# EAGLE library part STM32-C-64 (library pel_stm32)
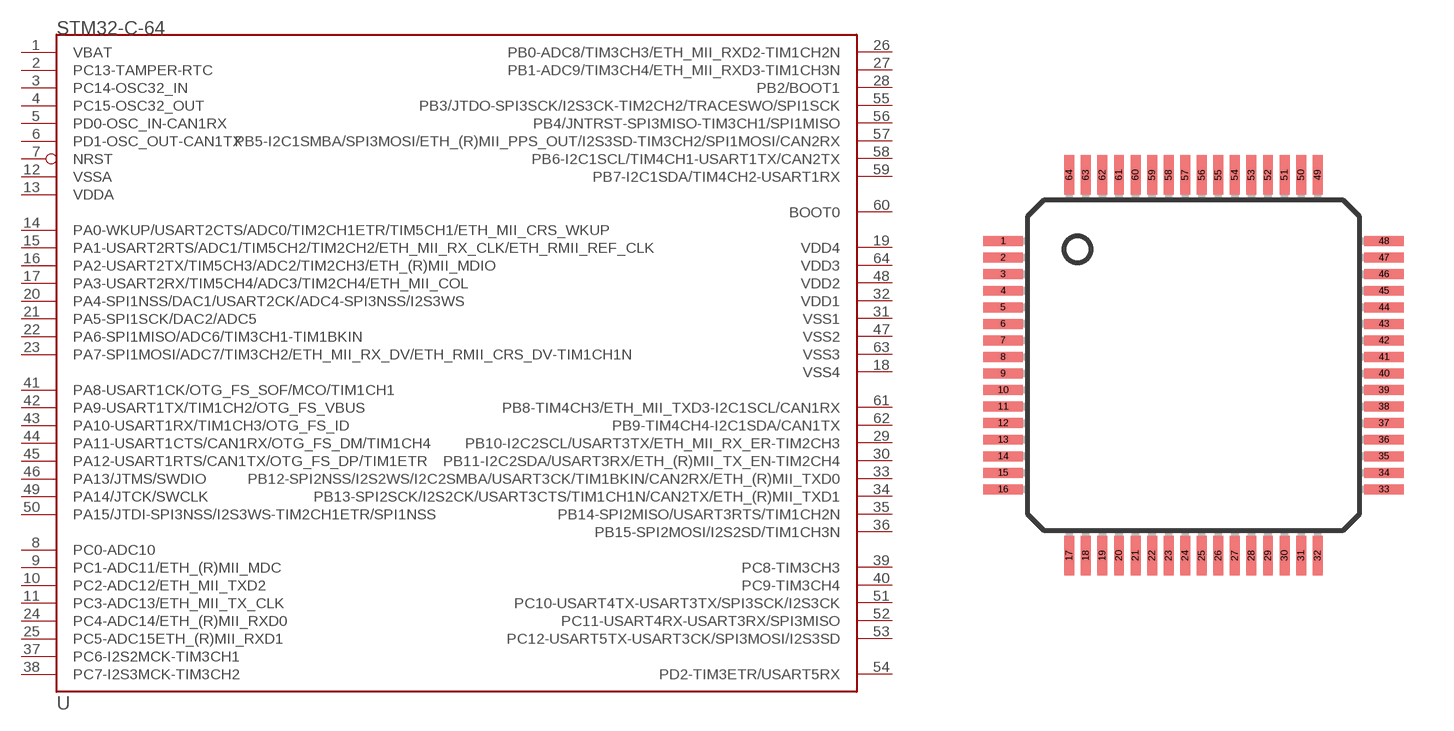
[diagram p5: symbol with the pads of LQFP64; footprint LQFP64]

Designator prefix U

## STM32-C-64  [LQFP64]
1  VBAT  sup
2  PC13-TAMPER-RTC
3  PC14-OSC32_IN
4  PC15-OSC32_OUT
5  PD0-OSC_IN-CAN1RX  in
6  PD1-OSC_OUT-CAN1TX  out
7  NRST
8  PC0-ADC10
9  PC1-ADC11/ETH_(R)MII_MDC
10  PC2-ADC12/ETH_MII_TXD2
11  PC3-ADC13/ETH_MII_TX_CLK
12  VSSA  sup
13  VDDA  sup
14  PA0-WKUP/USART2CTS/ADC0/TIM2CH1ETR/TIM5CH1/ETH_MII_CRS_WKUP
15  PA1-USART2RTS/ADC1/TIM5CH2/TIM2CH2/ETH_MII_RX_CLK/ETH_RMII_REF_CLK
16  PA2-USART2TX/TIM5CH3/ADC2/TIM2CH3/ETH_(R)MII_MDIO
17  PA3-USART2RX/TIM5CH4/ADC3/TIM2CH4/ETH_MII_COL
18  VSS4
19  VDD4
20  PA4-SPI1NSS/DAC1/USART2CK/ADC4-SPI3NSS/I2S3WS
21  PA5-SPI1SCK/DAC2/ADC5
22  PA6-SPI1MISO/ADC6/TIM3CH1-TIM1BKIN
23  PA7-SPI1MOSI/ADC7/TIM3CH2/ETH_MII_RX_DV/ETH_RMII_CRS_DV-TIM1CH1N
24  PC4-ADC14/ETH_(R)MII_RXD0
25  PC5-ADC15ETH_(R)MII_RXD1
26  PB0-ADC8/TIM3CH3/ETH_MII_RXD2-TIM1CH2N
27  PB1-ADC9/TIM3CH4/ETH_MII_RXD3-TIM1CH3N
28  PB2/BOOT1
29  PB10-I2C2SCL/USART3TX/ETH_MII_RX_ER-TIM2CH3
30  PB11-I2C2SDA/USART3RX/ETH_(R)MII_TX_EN-TIM2CH4
31  VSS1  sup
32  VDD1  sup
33  PB12-SPI2NSS/I2S2WS/I2C2SMBA/USART3CK/TIM1BKIN/CAN2RX/ETH_(R)MII_TXD0
34  PB13-SPI2SCK/I2S2CK/USART3CTS/TIM1CH1N/CAN2TX/ETH_(R)MII_TXD1
35  PB14-SPI2MISO/USART3RTS/TIM1CH2N
36  PB15-SPI2MOSI/I2S2SD/TIM1CH3N
37  PC6-I2S2MCK-TIM3CH1
38  PC7-I2S3MCK-TIM3CH2
39  PC8-TIM3CH3
40  PC9-TIM3CH4
41  PA8-USART1CK/OTG_FS_SOF/MCO/TIM1CH1
42  PA9-USART1TX/TIM1CH2/OTG_FS_VBUS
43  PA10-USART1RX/TIM1CH3/OTG_FS_ID
44  PA11-USART1CTS/CAN1RX/OTG_FS_DM/TIM1CH4
45  PA12-USART1RTS/CAN1TX/OTG_FS_DP/TIM1ETR
46  PA13/JTMS/SWDIO
47  VSS2  sup
48  VDD2  sup
49  PA14/JTCK/SWCLK
50  PA15/JTDI-SPI3NSS/I2S3WS-TIM2CH1ETR/SPI1NSS
51  PC10-USART4TX-USART3TX/SPI3SCK/I2S3CK
52  PC11-USART4RX-USART3RX/SPI3MISO
53  PC12-USART5TX-USART3CK/SPI3MOSI/I2S3SD
54  PD2-TIM3ETR/USART5RX
55  PB3/JTDO-SPI3SCK/I2S3CK-TIM2CH2/TRACESWO/SPI1SCK
56  PB4/JNTRST-SPI3MISO-TIM3CH1/SPI1MISO
57  PB5-I2C1SMBA/SPI3MOSI/ETH_(R)MII_PPS_OUT/I2S3SD-TIM3CH2/SPI1MOSI/CAN2RX
58  PB6-I2C1SCL/TIM4CH1-USART1TX/CAN2TX
59  PB7-I2C1SDA/TIM4CH2-USART1RX
60  BOOT0  in
61  PB8-TIM4CH3/ETH_MII_TXD3-I2C1SCL/CAN1RX
62  PB9-TIM4CH4-I2C1SDA/CAN1TX
63  VSS3  sup
64  VDD3  sup

## Footprint LQFP64 (pad centres in mm)
Based on STM PCB landpattern recomendation
smd 1.2 x 0.3: 1 -5.75,3.75; 2 -5.75,3.25; 3 -5.75,2.75; 4 -5.75,2.25; 5 -5.75,1.75; 6 -5.75,1.25; 7 -5.75,0.75; 8 -5.75,0.25; 9 -5.75,-0.25; 10 -5.75,-0.75; 11 -5.75,-1.25; 12 -5.75,-1.75; 13 -5.75,-2.25; 14 -5.75,-2.75; 15 -5.75,-3.25; 16 -5.75,-3.75; 33 5.75,-3.75; 34 5.75,-3.25; 35 5.75,-2.75; 36 5.75,-2.25; 37 5.75,-1.75; 38 5.75,-1.25; 39 5.75,-0.75; 40 5.75,-0.25; 41 5.75,0.25; 42 5.75,0.75; 43 5.75,1.25; 44 5.75,1.75; 45 5.75,2.25; 46 5.75,2.75; 47 5.75,3.25; 48 5.75,3.75
smd 0.3 x 1.2: 17 -3.75,-5.75; 18 -3.25,-5.75; 19 -2.75,-5.75; 20 -2.25,-5.75; 21 -1.75,-5.75; 22 -1.25,-5.75; 23 -0.75,-5.75; 24 -0.25,-5.75; 25 0.25,-5.75; 26 0.75,-5.75; 27 1.25,-5.75; 28 1.75,-5.75; 29 2.25,-5.75; 30 2.75,-5.75; 31 3.25,-5.75; 32 3.75,-5.75; 49 3.75,5.75; 50 3.25,5.75; 51 2.75,5.75; 52 2.25,5.75; 53 1.75,5.75; 54 1.25,5.75; 55 0.75,5.75; 56 0.25,5.75; 57 -0.25,5.75; 58 -0.75,5.75; 59 -1.25,5.75; 60 -1.75,5.75; 61 -2.25,5.75; 62 -2.75,5.75; 63 -3.25,5.75; 64 -3.75,5.75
